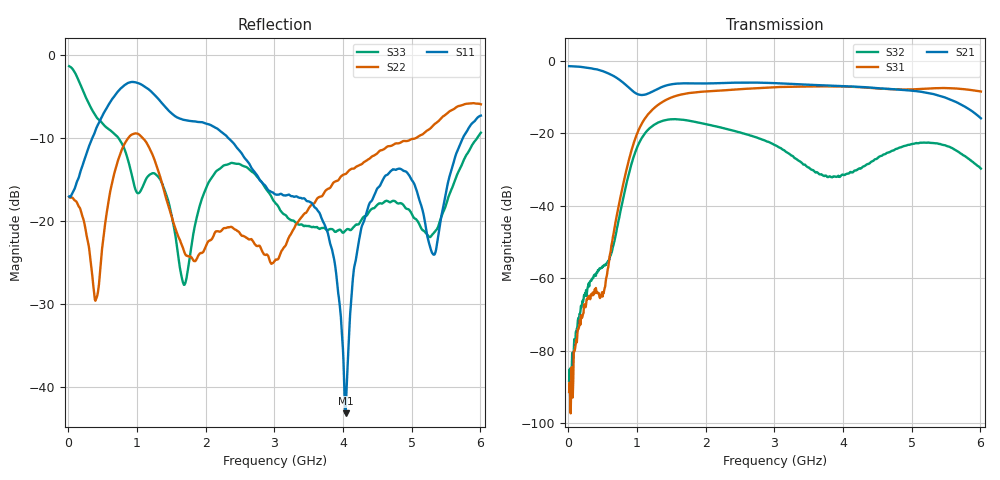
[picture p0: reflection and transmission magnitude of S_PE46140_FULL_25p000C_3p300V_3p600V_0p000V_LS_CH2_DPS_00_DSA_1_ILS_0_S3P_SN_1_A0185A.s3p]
! Device ID: PE46140_FULL
! File Path: z:\PE46140\MajorStates\25p000C\3p300\LS_CH2_DPS_00_DSA_1_ILS_0\PE46140_FULL_25p000C_3p300V_3p600V_0p000V_LS_CH2_DPS_00_DSA_1_ILS_0_S3P_SN_1_A0185A.s3p
! Serial: 1
! Lot: A0185A
! Temp: 25.000C
! VDD: 3.300
! VSS: 0.000
! Control_Hi: 3.600
! Control_Lo: 0.000
! Logic State: LS_CH2_DPS_00_DSA_1_ILS_0
! Port 1: RFIN
! Port 2: RFOUT1
! Port 3: RFOUT2
! ThroughPath:1-3
! IDD: 0.0003148759
! ISS: -1.694e-007
! Comment:
#  Hz  S  RI  R  50
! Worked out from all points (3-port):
!   801 points, 10 MHz to 6.01 GHz, reference 50 ohm
!   strongest paths, dB at 10 MHz, 1.51 GHz, 3.01 GHz, 4.51 GHz, 6.01 GHz:
!     S21: -1.5, -6.5, -6.2, -7.6, -15.9
!     S31: -91.3, -10.1, -7.3, -7.7, -8.5
!     S32: -88.3, -16.1, -23.3, -26.7, -29.8
!   lowest |S11| = -43.2 dB at 4.037 GHz (marker M1), VSWR 1.01, Z = 49.3 + j0.163 ohm
!   |S11| at or under -10 dB: start of sweep to 346.1 MHz; 2.333 GHz to 5.746 GHz (3.413 GHz wide, 84.5 % of centre)
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1e7  0.1402 -0.0108  0.8421 -0.0244  1.89e-05 2.15e-06
     0.8417 -0.0244  0.1399 -0.00677  -1.72e-05 3.55e-05
     -1.33e-05 2.36e-05  3.65e-05 1.23e-05  0.858 -0.0813
3.55e8  -0.016 -0.3219  0.4592 -0.6283  -0.000536 -0.000256
        0.4593 -0.6262  -0.00911 -0.0426  -0.000126 0.000957
        -0.00057 -0.000283  -0.00012 0.00101  -0.4111 -0.2087
1.165e9  -0.5853 0.2235  -0.205 -0.2877  -0.1824 -0.0264
         -0.2052 -0.2884  0.2134 -0.1871  -0.00235 0.1128
         -0.1827 -0.0267  -0.00248 0.1128  0.1558 0.1042
1.9825e9  -0.1842 0.3449  -0.4182 0.2483  0.3716 -0.0565
          -0.4183 0.2481  0.0621 -0.0261  -0.134 -0.0159
          0.3719 -0.0565  -0.134 -0.0159  0.0442 0.1432
3.01e9  0.0222 0.1435  0.4085 0.2722  -0.3744 -0.2147
        0.4083 0.273  -0.0577 -0.00142  0.0612 -0.0307
        -0.3748 -0.215  0.0612 -0.031  0.124 -0.0362
3.7525e9  0.0234 0.0872  0.2864 -0.3557  -0.2391 0.3734
          0.287 -0.3555  0.0754 0.1338  -0.0166 0.0202
          -0.2388 0.3735  -0.0165 0.0202  0.0886 -0.00927
4.0375e9  -0.0067 0.00165  0.0428 -0.4428  -0.00237 0.4403
          0.0433 -0.443  0.1394 0.1325  0.0228 0.0146
          -0.00125 0.44  0.0229 0.0146  0.0869 -0.0113
4.39e9  -0.1067 -0.072  -0.2578 -0.3407  0.2638 0.331
        -0.2579 -0.3409  0.2178 0.0979  0.0132 -0.0363
        0.2642 0.3303  0.0132 -0.0362  0.1122 -0.0241
5.3275e9  -0.0411 -0.0473  -0.114 0.3256  0.3067 -0.2826
          -0.1148 0.3258  0.3806 -0.0362  0.0101 0.0725
          0.3064 -0.2829  0.0101 0.0722  0.0846 0.0104
6.01e9  -0.3034 -0.3097  0.1529 0.048  -0.1912 -0.3228
        0.1536 0.0483  0.2471 -0.4429  0.0274 -0.0177
        -0.1927 -0.3236  0.0272 -0.0178  0.3195 0.121
